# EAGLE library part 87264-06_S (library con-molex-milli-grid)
RECEPTACAL
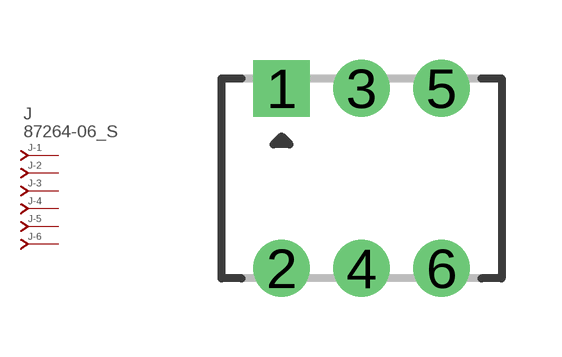
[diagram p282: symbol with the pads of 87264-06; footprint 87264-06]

Designator prefix J; gates -1=J-NV -2=J-N -3=J-N -4=J-N -5=J-N -6=J-N

## 87264-06_S  [87264-06]
1  -1:J  pas
2  -2:J  pas
3  -3:J  pas
4  -4:J  pas
5  -5:J  pas
6  -6:J  pas

## Footprint 87264-06 (pad centres in mm)
RECEPTACAL Dual Row, Side Entry
drill 0.914 square: 1 -2,2.25
drill 0.914: 2 -2,-2.25; 3 0,2.25; 4 0,-2.25; 5 2,2.25; 6 2,-2.25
